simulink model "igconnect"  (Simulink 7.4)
settings: Solver=ode45  StartTime=0  StopTime=30  MaxStep=1e-3  RelTol=1e-3
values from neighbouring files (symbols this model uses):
  wo = 2*pi*freq0    [calc0.m]    (also in IMabc2.m = 376.991118431; imabcparam.m = 376.991118431; IMabcrun0.m = 376.991118431; IMabcrun1.m = 376.991118431)
undefined symbols (not defined in the file or in its folder): fro, fso, gamo, vro, vso, wmo
libraries: simulink_extras x1

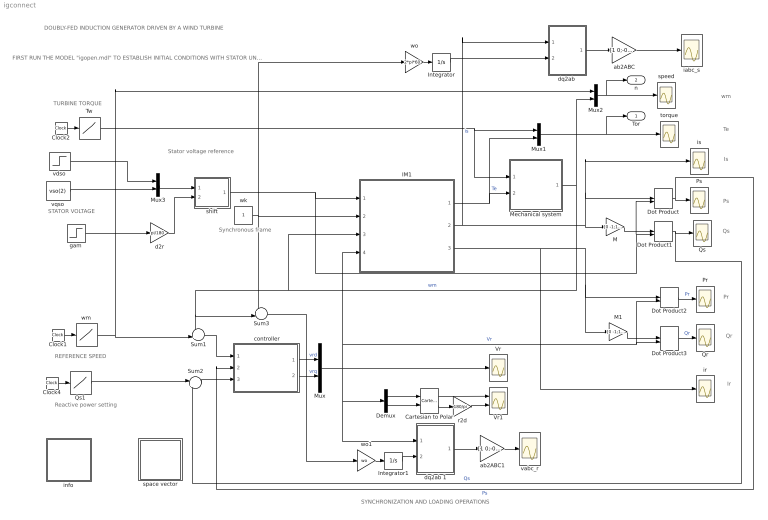
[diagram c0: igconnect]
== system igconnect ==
  note: Reactive power setting
  note: TURBINE TORQUE
  note: REFERENCE SPEED
  note: Synchronous frame
  note: Stator voltage reference
  note: DOUBLY-FED INDUCTION GENERATOR DRIVEN BY A WIND TURBINE
  note: STATOR VOLTAGE
  note: SYNCHRONIZATION AND LOADING OPERATIONS
  note: FIRST RUN THE MODEL "igopen.mdl" TO ESTABLISH INITIAL CONDITIONS WITH STATOR UNCONNECTED TO GRID
  note: Pr
  note: Qr
  note: Ps
  note: Qs
  note: Is
  note: Ir
  note: Te
  note: wm
  " controller" : Subsystem  mask{Kpn=8, Kin=8, Kpt=2, Kit=1, KpQ=1, KiQ=10, sat=2}
      mask prompts: Kpn "Proportional gain of speed loop"; Kin "Integral gain of speed loop"; Kpt "Proportional gain of torque loop"; Kit "Integral gain of torque loop"; KpQ "Proportional gain of Qs loop"; KiQ "Integral gain of Qs loop"; sat "Saturation limit [pu]"
      mask help: PI controllers for speed, Ps, and Qs
  Cartesian to Polar : simulink_extras/Transformations/Cartesian to Polar  SystemSampleTime=-1
  Clock1 : Clock
  Clock2 : Clock
  Clock4 : Clock
  Demux : Demux  Outputs=2
  Dot Product{,1..3} (4 alike) : DotProduct  OutDataType=fixdt(1, 16)  OutScaling=2^-10
  IM1 : Subsystem  mask{Rs=0.05, Lsl=0.1, Rr=0.02, Lm=5, Lrl=0.1, wo=wo}
      mask prompts: Rs "Stator resistance [pu]"; Lsl "Stator leakage inductance [pu]"; Rr "Rotor resistance [pu]"; Lm "Magnetizing inductance [pu]"; Lrl "Rotor leakage inductance [pu]"; wo "base frequency [rad/s]"
  Integrator : Integrator
  Integrator1 : Integrator
  M : Gain  Gain=[0 -1;1 0]  Multiplication=Matrix(K*u)  ParameterDataType=sfix(16)  ParameterScaling=2^0  OutDataType=sfix(16)  OutScaling=2^0
  M1 : Gain  Gain=[0 -1;1 0]  Multiplication=Matrix(K*u)  ParameterDataType=sfix(16)  ParameterScaling=2^0  OutDataType=sfix(16)  OutScaling=2^0
  Mechanical system : Subsystem  mask{Hw=2.5, Hg=0.5, Km=.4}
      mask prompts: Hw "Turbine inertia constant [s]"; Hg "Generator inertia constant [s]"; Km "Shaft compliance constant [pu/rad]"
  Mux{,1..3} (4 alike) : Mux  Inputs=2
  Pr : Scope
  Ps : Scope
  Qr : Scope
  Qs : Scope
  Qs1 : Lookup  InputValues=[0 20 25 30]  Table="[0 0  -.5 -.5]"  OutDataType=sfix(16)  OutScaling=2^0
  Sum1 : Sum  Inputs=-+|  OutDataType=sfix(16)  OutScaling=2^0
  Sum2 : Sum  Inputs=|+-  OutDataType=sfix(16)  OutScaling=2^0
  Sum3 : Sum  Inputs=+-|  OutDataType=sfix(16)  OutScaling=2^0
  Tw : Lookup  InputValues="[0  10 15 30 ]"  Table="[0 0  -1 -1]"  OutDataType=sfix(16)  OutScaling=2^0
  Vr : Scope
  Vr1 : Scope  NumInputPorts=2
  ab2ABC : Gain  Gain=[1 0;-0.5 sqrt(3)/2;-0.5 -sqrt(3)/2]  Multiplication=Matrix(K*u)  ParameterDataType=sfix(16)  ParameterScaling=2^0  OutDataType=sfix(16)  OutScaling=2^0
  ab2ABC1 : Gain  Gain=[1 0;-0.5 sqrt(3)/2;-0.5 -sqrt(3)/2]  Multiplication=Matrix(K*u)  ParameterDataType=sfix(16)  ParameterScaling=2^0  OutDataType=sfix(16)  OutScaling=2^0
  d2r : Gain  Gain=pi/180  Multiplication=Matrix(K*u)  ParameterDataType=sfix(16)  ParameterScaling=2^0  OutDataType=sfix(16)  OutScaling=2^0
  "dq2ab " : Subsystem
  dq2ab 1 : Subsystem
  gam : Step  Before=gamo  After=0  SampleTime=0
  iabc_s : Scope
  info : Subsystem
  ir : Scope
  is : Scope
  r2d : Gain  Gain=180/pi  Multiplication=Matrix(K*u)  ParameterDataType=sfix(16)  ParameterScaling=2^0  OutDataType=sfix(16)  OutScaling=2^0
  shift : Subsystem
  space vector : Subsystem
  speed : Scope
  torque : Scope
  vabc_r : Scope
  vdso : Step  Before=vso(1)  After=1.0  SampleTime=0
  vqso : Constant  Value=vso(2)  OutDataType=sfix(16)  OutScaling=2^0
  wk : Constant  OutDataType=sfix(16)  OutScaling=2^0
  wm : Lookup  InputValues=[0 20 20.01 30 ]  Table=[wmo wmo wmo wmo]  OutDataType=sfix(16)  OutScaling=2^0
  wo : Gain  Gain=2*pi*60  ParameterDataType=sfix(16)  ParameterScaling=2^0  OutDataType=sfix(16)  OutScaling=2^0
  wo1 : Gain  Gain=wo  ParameterDataType=sfix(16)  ParameterScaling=2^0  OutDataType=sfix(16)  OutScaling=2^0
  Tor : Outport
  n : Outport  Port=2
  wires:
  wk/1 -> IM1/2(wk), wo/1, Sum3/1
  Dot Product/1 -> Ps/1, " controller"/2(Ps)  "Ps"
  M/1 -> Dot Product1/1
  IM1/1(Te) -> Mechanical system/2(Te), Mux1/2  "Te"
  Clock2/1 -> Tw/1
  " controller"/1(vrd) -> Mux/1  "vrd"
  Dot Product1/1 -> Qs/1, Sum2/2  "Qs"
  Mux1/1 -> torque/1, Tor/1
  IM1/2(is) -> M/1, Dot Product/1, is/1, "dq2ab "/1(dq)  "is"
  Dot Product2/1 -> Pr/1  "Pr"
  M1/1 -> Dot Product3/1
  Dot Product3/1 -> Qr/1  "Qr"
  IM1/3(ir) -> M1/1, Dot Product2/1, ir/1
  Mechanical system/1(wm) -> IM1/3(wm), Sum1/1, Sum3/2, Mux2/2  "wm"
  Sum1/1 -> " controller"/1(wmer)
  wm/1 -> Sum1/2, Mux2/1
  Mux2/1 -> speed/1, n/1
  Clock1/1 -> wm/1
  shift/1(vs) -> Dot Product/2, Dot Product1/2, IM1/1(vs)
  Demux/1 -> Cartesian to Polar/1
  Demux/2 -> Cartesian to Polar/2
  Cartesian to Polar/1 -> Vr1/1
  Cartesian to Polar/2 -> r2d/1
  r2d/1 -> Vr1/2
  Mux/1 -> IM1/4(vr), Dot Product3/2, Dot Product2/2, Vr/1, Demux/1, dq2ab 1/1(dq)  "Vr"
  d2r/1 -> shift/2(gama)
  Mux3/1 -> shift/1(vso)
  vqso/1 -> Mux3/2
  vdso/1 -> Mux3/1
  "dq2ab "/1(ab) -> ab2ABC/1
  ab2ABC/1 -> iabc_s/1
  wo/1 -> Integrator/1
  Tw/1 -> Mux1/1, Mechanical system/1(Tw)
  Integrator/1 -> "dq2ab "/2(thetas)
  Sum2/1 -> " controller"/3(Qser)
  " controller"/2(vrq) -> Mux/2  "vrq"
  Clock4/1 -> Qs1/1
  Qs1/1 -> Sum2/1
  gam/1 -> d2r/1
  dq2ab 1/1(ab) -> ab2ABC1/1
  ab2ABC1/1 -> vabc_r/1
  wo1/1 -> Integrator1/1
  Integrator1/1 -> dq2ab 1/2(thetas)
  Sum3/1 -> wo1/1

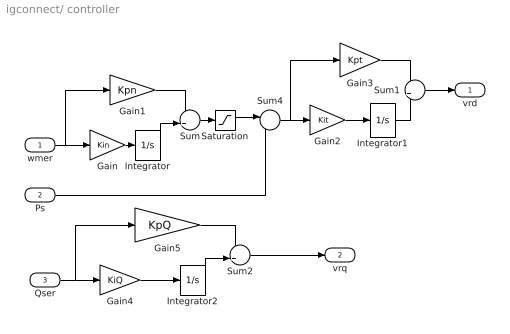
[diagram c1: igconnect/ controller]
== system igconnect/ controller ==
  wmer : Inport  OutDataType=sfix(16)  OutScaling=2^0
  Ps : Inport  Port=2  OutDataType=sfix(16)  OutScaling=2^0
  Qser : Inport  Port=3  OutDataType=sfix(16)  OutScaling=2^0
  Gain : Gain  Gain=Kin  ParameterDataType=sfix(16)  ParameterScaling=2^0  OutDataType=sfix(16)  OutScaling=2^0
  Gain1 : Gain  Gain=Kpn  ParameterDataType=sfix(16)  ParameterScaling=2^0  OutDataType=sfix(16)  OutScaling=2^0
  Gain2 : Gain  Gain=Kit  ParameterDataType=sfix(16)  ParameterScaling=2^0  OutDataType=sfix(16)  OutScaling=2^0
  Gain3 : Gain  Gain=Kpt  ParameterDataType=sfix(16)  ParameterScaling=2^0  OutDataType=sfix(16)  OutScaling=2^0
  Gain4 : Gain  Gain=KiQ  ParameterDataType=sfix(16)  ParameterScaling=2^0  OutDataType=sfix(16)  OutScaling=2^0
  Gain5 : Gain  Gain=KpQ  ParameterDataType=sfix(16)  ParameterScaling=2^0  OutDataType=sfix(16)  OutScaling=2^0
  Integrator : Integrator  LimitOutput=on  UpperSaturationLimit=sat  LowerSaturationLimit=-sat
  Integrator1 : Integrator  InitialCondition=vro(1)  UpperSaturationLimit=sat  LowerSaturationLimit=-sat
  Integrator2 : Integrator  InitialCondition=vro(2)  UpperSaturationLimit=sat  LowerSaturationLimit=-sat
  Saturation : Saturate  UpperLimit=sat  LowerLimit=-sat
  Sum : Sum  OutDataType=sfix(16)  OutScaling=2^0
  Sum1 : Sum  OutDataType=sfix(16)  OutScaling=2^0
  Sum2 : Sum  OutDataType=sfix(16)  OutScaling=2^0
  Sum4 : Sum  Inputs=|-+  OutDataType=sfix(16)  OutScaling=2^0
  vrd : Outport  InitialOutput=0
  vrq : Outport  Port=2  InitialOutput=0
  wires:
  Sum/1 -> Saturation/1
  wmer/1 -> Gain1/1, Gain/1
  Gain/1 -> Integrator/1
  Gain1/1 -> Sum/1
  Integrator/1 -> Sum/2
  Sum1/1 -> vrd/1
  Sum4/1 -> Gain2/1, Gain3/1
  Gain2/1 -> Integrator1/1
  Gain3/1 -> Sum1/1
  Integrator1/1 -> Sum1/2
  Saturation/1 -> Sum4/1
  Sum2/1 -> vrq/1
  Qser/1 -> Gain5/1, Gain4/1
  Gain4/1 -> Integrator2/1
  Gain5/1 -> Sum2/1
  Integrator2/1 -> Sum2/2
  Ps/1 -> Sum4/2

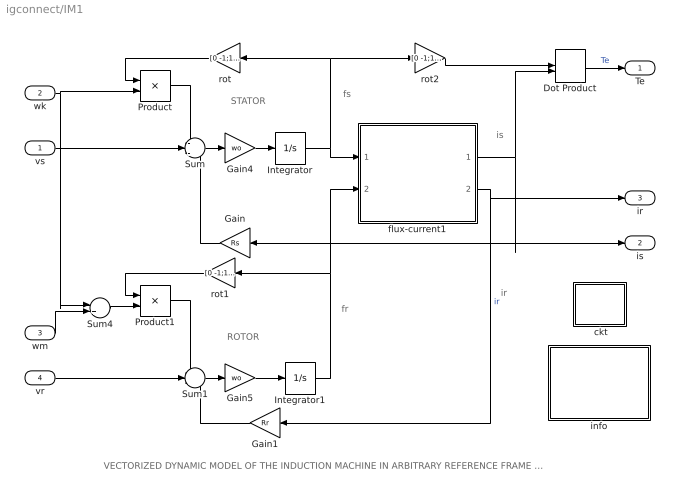
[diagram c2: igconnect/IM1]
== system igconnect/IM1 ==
  note: ROTOR
  note: STATOR
  note: fs
  note: fr
  note: is
  note: VECTORIZED DYNAMIC MODEL OF THE INDUCTION MACHINE IN ARBITRARY REFERENCE FRAME (per unit formulation)
  note: ir
  vs : Inport  OutDataType=sfix(16)  OutScaling=2^0
  wk : Inport  Port=2  OutDataType=sfix(16)  OutScaling=2^0
  wm : Inport  Port=3  OutDataType=sfix(16)  OutScaling=2^0
  vr : Inport  Port=4  OutDataType=sfix(16)  OutScaling=2^0
  " ckt" : Subsystem
  Dot Product : DotProduct  OutDataType=fixdt(1, 16)  OutScaling=2^-10
  Gain : Gain  Gain=Rs  ParameterDataType=sfix(16)  ParameterScaling=2^0  OutDataType=sfix(16)  OutScaling=2^0
  Gain1 : Gain  Gain=Rr  ParameterDataType=sfix(16)  ParameterScaling=2^0  OutDataType=sfix(16)  OutScaling=2^0
  Gain4 : Gain  Gain=wo  ParameterDataType=sfix(16)  ParameterScaling=2^0  OutDataType=sfix(16)  OutScaling=2^0
  Gain5 : Gain  Gain=wo  ParameterDataType=sfix(16)  ParameterScaling=2^0  OutDataType=sfix(16)  OutScaling=2^0
  Integrator : Integrator  InitialCondition=fso
  Integrator1 : Integrator  InitialCondition=fro
  Product : Product  OutDataType=sfix(16)  OutScaling=2^0
  Product1 : Product  OutDataType=sfix(16)  OutScaling=2^0
  Sum : Sum  Inputs=-+-  OutDataType=sfix(16)  OutScaling=2^0
  Sum1 : Sum  Inputs=-+-  OutDataType=sfix(16)  OutScaling=2^0
  Sum4 : Sum  Inputs=|+-  OutDataType=sfix(16)  OutScaling=2^0
  flux-current1 : Subsystem
  info : Subsystem
  rot : Gain  Gain=[0 -1;1 0]  Multiplication=Matrix(K*u)  ParameterDataType=sfix(16)  ParameterScaling=2^0  OutDataType=sfix(16)  OutScaling=2^0
  rot1 : Gain  Gain=[0 -1;1 0]  Multiplication=Matrix(K*u)  ParameterDataType=sfix(16)  ParameterScaling=2^0  OutDataType=sfix(16)  OutScaling=2^0
  rot2 : Gain  Gain=[0 -1;1 0]  Multiplication=Matrix(K*u)  ParameterDataType=sfix(16)  ParameterScaling=2^0  OutDataType=sfix(16)  OutScaling=2^0
  Te : Outport
  is : Outport  Port=2
  ir : Outport  Port=3
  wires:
  Gain/1 -> Sum/3
  Gain1/1 -> Sum1/3
  flux-current1/2(ir) -> Gain1/1, ir/1  "ir"
  Integrator/1 -> flux-current1/1(fs), rot/1, rot2/1
  Integrator1/1 -> flux-current1/2(fr), rot1/1
  Product1/1 -> Sum1/1
  rot1/1 -> Product1/1
  Product/1 -> Sum/1
  rot/1 -> Product/1
  rot2/1 -> Dot Product/1
  Sum4/1 -> Product1/2
  Sum/1 -> Gain4/1
  Gain4/1 -> Integrator/1
  Sum1/1 -> Gain5/1
  Gain5/1 -> Integrator1/1
  flux-current1/1(is) -> Gain/1, is/1, Dot Product/2
  Dot Product/1 -> Te/1  "Te"
  vs/1 -> Sum/2
  wk/1 -> Product/2, Sum4/1
  wm/1 -> Sum4/2
  vr/1 -> Sum1/2

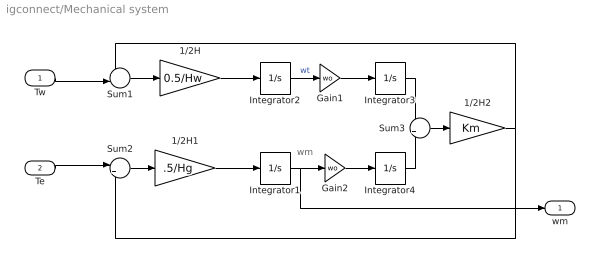
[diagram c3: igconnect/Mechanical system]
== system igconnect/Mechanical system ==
  note: wm
  Tw : Inport  OutDataType=sfix(16)  OutScaling=2^0
  Te : Inport  Port=2  OutDataType=sfix(16)  OutScaling=2^0
  1/2H : Gain  Gain=0.5/Hw  ParameterDataType=sfix(16)  ParameterScaling=2^0  OutDataType=sfix(16)  OutScaling=2^0
  1/2H1 : Gain  Gain=.5/Hg  ParameterDataType=sfix(16)  ParameterScaling=2^0  OutDataType=sfix(16)  OutScaling=2^0
  1/2H2 : Gain  Gain=Km  ParameterDataType=sfix(16)  ParameterScaling=2^0  OutDataType=sfix(16)  OutScaling=2^0
  Gain1 : Gain  Gain=wo  ParameterDataType=sfix(16)  ParameterScaling=2^0  OutDataType=sfix(16)  OutScaling=2^0
  Gain2 : Gain  Gain=wo  ParameterDataType=sfix(16)  ParameterScaling=2^0  OutDataType=sfix(16)  OutScaling=2^0
  Integrator1 : Integrator  InitialCondition=wmo
  Integrator2 : Integrator  InitialCondition=wmo
  Integrator3 : Integrator
  Integrator4 : Integrator
  Sum1 : Sum  Inputs=+-|  OutDataType=sfix(16)  OutScaling=2^0
  Sum2 : Sum  Inputs=|+-  OutDataType=sfix(16)  OutScaling=2^0
  Sum3 : Sum  Inputs=-+  OutDataType=sfix(16)  OutScaling=2^0
  wm : Outport
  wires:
  Tw/1 -> Sum1/2
  Sum1/1 -> 1/2H/1
  Te/1 -> Sum2/1
  1/2H/1 -> Integrator2/1
  Sum2/1 -> 1/2H1/1
  1/2H1/1 -> Integrator1/1
  Integrator3/1 -> Sum3/1
  Sum3/1 -> 1/2H2/1
  1/2H2/1 -> Sum1/1, Sum2/2
  Gain1/1 -> Integrator3/1
  Integrator2/1 -> Gain1/1  "wt"
  Gain2/1 -> Integrator4/1
  Integrator4/1 -> Sum3/2
  Integrator1/1 -> Gain2/1, wm/1

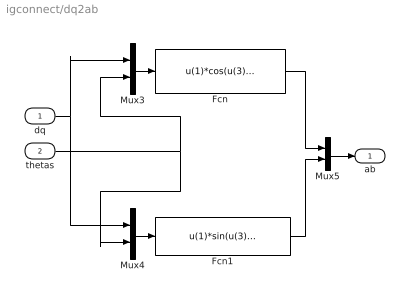
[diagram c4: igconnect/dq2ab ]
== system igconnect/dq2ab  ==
  dq : Inport  OutDataType=sfix(16)  OutScaling=2^0
  thetas : Inport  Port=2  OutDataType=sfix(16)  OutScaling=2^0
  Fcn : Fcn  Expr=u(1)*cos(u(3))-u(2)*sin(u(3))
  Fcn1 : Fcn  Expr=u(1)*sin(u(3))+u(2)*cos(u(3))
  Mux3 : Mux  Inputs=2
  Mux4 : Mux  Inputs=2
  Mux5 : Mux  Inputs=2
  ab : Outport
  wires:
  Mux3/1 -> Fcn/1
  Mux4/1 -> Fcn1/1
  dq/1 -> Mux3/1, Mux4/1
  thetas/1 -> Mux3/2, Mux4/2
  Fcn1/1 -> Mux5/2
  Fcn/1 -> Mux5/1
  Mux5/1 -> ab/1

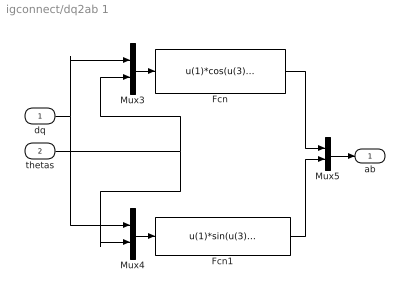
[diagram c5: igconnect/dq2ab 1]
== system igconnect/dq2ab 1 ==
  dq : Inport  OutDataType=sfix(16)  OutScaling=2^0
  thetas : Inport  Port=2  OutDataType=sfix(16)  OutScaling=2^0
  Fcn : Fcn  Expr=u(1)*cos(u(3))-u(2)*sin(u(3))
  Fcn1 : Fcn  Expr=u(1)*sin(u(3))+u(2)*cos(u(3))
  Mux3 : Mux  Inputs=2
  Mux4 : Mux  Inputs=2
  Mux5 : Mux  Inputs=2
  ab : Outport
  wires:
  Mux3/1 -> Fcn/1
  Mux4/1 -> Fcn1/1
  dq/1 -> Mux3/1, Mux4/1
  thetas/1 -> Mux3/2, Mux4/2
  Fcn1/1 -> Mux5/2
  Fcn/1 -> Mux5/1
  Mux5/1 -> ab/1

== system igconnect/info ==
  note: The induction machine is modeled in vectorized form in the synchronous frame associated with the stator voltage space vector. The dq components of the injected rotor voltage Vr, at slip frequency wr, are derived from PI controllers; vrd is the output of a cascade arrangement of speed and Ps controllers; vrq is derived from a Qs controller. The mechanical system is modeled as two inertias coupled by means of a flexible shaft. The whole system is described by parameters expressed in per unit. The machine representations are based on the motor convention; consequently, in the generator mode of operation, such quantities as Ps, Qs, Tw, Te are negative (with wm>0) while Pr is positive for subsynchronous operation and negative for oversynchronous mode. Before running this model, must be run first to establish the initial conditions representing the generator disconnected from the grid. The present model simulates the connection to the grid followed by the active and reactive loading of the generator.
  note: Doubly-Fed Induction Generator driven by a Wind Turbine

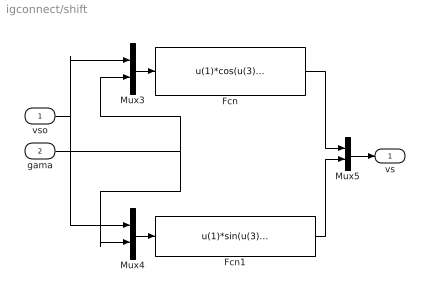
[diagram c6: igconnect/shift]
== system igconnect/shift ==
  vso : Inport  OutDataType=sfix(16)  OutScaling=2^0
  gama : Inport  Port=2  OutDataType=sfix(16)  OutScaling=2^0
  Fcn : Fcn  Expr=u(1)*cos(u(3))-u(2)*sin(u(3))
  Fcn1 : Fcn  Expr=u(1)*sin(u(3))+u(2)*cos(u(3))
  Mux3 : Mux  Inputs=2
  Mux4 : Mux  Inputs=2
  Mux5 : Mux  Inputs=2
  vs : Outport
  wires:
  Mux5/1 -> vs/1
  Fcn/1 -> Mux5/1
  Fcn1/1 -> Mux5/2
  gama/1 -> Mux4/2, Mux3/2
  vso/1 -> Mux4/1, Mux3/1
  Mux4/1 -> Fcn1/1
  Mux3/1 -> Fcn/1

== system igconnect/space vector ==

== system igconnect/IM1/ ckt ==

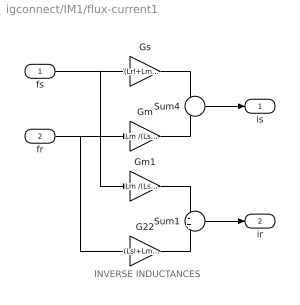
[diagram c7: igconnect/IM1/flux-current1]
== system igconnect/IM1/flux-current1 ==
  note: INVERSE INDUCTANCES
  fs : Inport  OutDataType=sfix(16)  OutScaling=2^0
  fr : Inport  Port=2  OutDataType=sfix(16)  OutScaling=2^0
  G22 : Gain  Gain=(Lsl+Lm )/(Lsl*Lrl+Lsl*Lm+Lrl*Lm)  ParameterDataType=sfix(16)  ParameterScaling=2^0  OutDataType=sfix(16)  OutScaling=2^0
  Gm : Gain  Gain=Lm /(Lsl*Lrl+Lsl*Lm+Lrl*Lm)  ParameterDataType=sfix(16)  ParameterScaling=2^0  OutDataType=sfix(16)  OutScaling=2^0
  Gm1 : Gain  Gain=Lm /(Lsl*Lrl+Lsl*Lm+Lrl*Lm)  ParameterDataType=sfix(16)  ParameterScaling=2^0  OutDataType=sfix(16)  OutScaling=2^0
  Gs : Gain  Gain=(Lrl+Lm) /(Lsl*Lrl+Lsl*Lm+Lrl*Lm)  ParameterDataType=sfix(16)  ParameterScaling=2^0  OutDataType=sfix(16)  OutScaling=2^0
  Sum1 : Sum  Inputs=-+  OutDataType=sfix(16)  OutScaling=2^0
  Sum4 : Sum  Inputs=+-  OutDataType=sfix(16)  OutScaling=2^0
  is : Outport
  ir : Outport  Port=2
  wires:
  fs/1 -> Gs/1, Gm1/1
  Gs/1 -> Sum4/1
  fr/1 -> Gm/1, G22/1
  Gm/1 -> Sum4/2
  Sum4/1 -> is/1
  Gm1/1 -> Sum1/1
  G22/1 -> Sum1/2
  Sum1/1 -> ir/1

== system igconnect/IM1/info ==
  note: Mathematical model of the induction machine. Space vector formulation in an arbitrary dq common reference frame. Per unit description.
  note: Electrical system equations: vs = Rs is + 1/wo (dfs/dt) + wk M(pi/2) fs vr = Rr ir + 1/wo (dfr/dt) + (wk - wm) M(pi/2) fr where the variables i, v, and f are 2-dimensional space vectors; for instance is = [ids iqs] and so forth, wk is the speed of the reference frame, wm the rotor speed, and M(pi/2)represents a 90o space rotator namely M(pi/2) = [0 -1;1 0] The flux linkage current relations are: fs = Ls is + Lm ir fr = Lm is + Lr ir where Ls =Lm +Lsl and Lr = Lm +Lrl Mechanical system equations: Te = 2H (dwm/dt ) + Bm wm + Tl where Te = fs (cross) is = M(pi/2) fs (dot) is = fds iqs - fqs ids = fs x is = M(pi/2) fs . is = ir x fr = Lm (ir x is) = Lm/Lr (fr x is) = 1/Lm' (fr x fs) Lm' =Lm c/(1-c) c = 1 - Lm^2/(Ls Lr)
